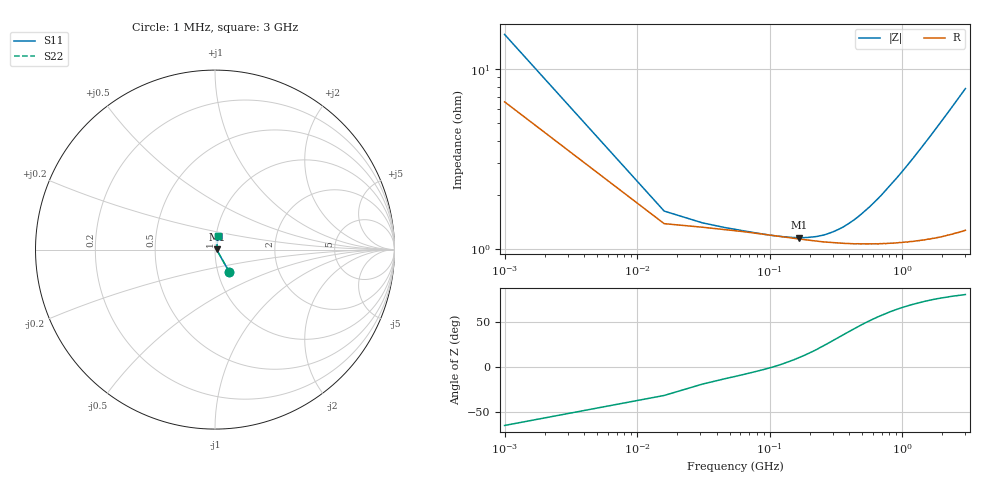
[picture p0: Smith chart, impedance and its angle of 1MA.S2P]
!Keysight Technologies,E4991B,MY54301043,A.02.04
!Date: Thu Nov 16 21:14:31 2023
!Data:
!Freq	S11	S21	S12	S22
# Hz S MA R 50
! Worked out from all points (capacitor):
!   201 points, 1 MHz to 3 GHz, reference 50 ohm
!   read as one part in series: C = 10.2 nF near 15.99 MHz
!   lowest |Z| = 1.16 ohm at 165.9 MHz (marker M1)
!   series resonance near 105.6 MHz, so ESL is about 220 pH
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1000000  0.1448 -57.4  0.9301 7.5  0.9301 7.5  0.1448 -57.4
1.5995e7  0.0161 -31.1  0.9863 0.5  0.9863 0.5  0.0161 -31.1
3.099e7  0.01387 -18.8  0.9869 0.3  0.9869 0.3  0.01387 -18.8
4.5985e7  0.01306 -12.9  0.9873 0.2  0.9873 0.2  0.01306 -12.9
6.098e7  0.01259 -8.8  0.9876 0.1  0.9876 0.1  0.01259 -8.8
7.5975e7  0.01225 -5.5  0.9878 0.1  0.9878 0.1  0.01225 -5.5
1.05965e8  0.01181 0.1  0.9882 -0.0  0.9882 -0.0  0.01181 0.1
1.35955e8  0.01158 5.3  0.9885 -0.1  0.9885 -0.1  0.01158 5.3
1.65945e8  0.01149 10.2  0.9887 -0.1  0.9887 -0.1  0.01149 10.2
2.25925e8  0.01167 19.2  0.989 -0.2  0.989 -0.2  0.01167 19.2
3.009e8  0.01239 29.1  0.9892 -0.3  0.9892 -0.3  0.01239 29.1
3.6088e8  0.01321 35.5  0.9893 -0.4  0.9893 -0.4  0.01321 35.5
5.1083e8  0.01592 47.4  0.9893 -0.7  0.9893 -0.7  0.01592 47.4
6.3079e8  0.01839 53.8  0.9892 -0.9  0.9892 -0.9  0.01839 53.8
7.8074e8  0.02169 59.4  0.9891 -1.1  0.9891 -1.1  0.02169 59.4
1.005665e9  0.0269 64.8  0.9889 -1.4  0.9889 -1.4  0.0269 64.8
1.245585e9  0.03261 68.5  0.9885 -1.8  0.9885 -1.8  0.03261 68.5
1.5005e9  0.03881 71.1  0.9881 -2.1  0.9881 -2.1  0.03881 71.1
1.725425e9  0.0444 72.7  0.9877 -2.5  0.9877 -2.5  0.0444 72.7
2.01033e9  0.05151 74.1  0.9871 -2.9  0.9871 -2.9  0.05151 74.1
2.505165e9  0.0641 75.5  0.9859 -3.6  0.9859 -3.6  0.0641 75.5
3e9  0.07678 76.2  0.9845 -4.3  0.9845 -4.3  0.07678 76.2
